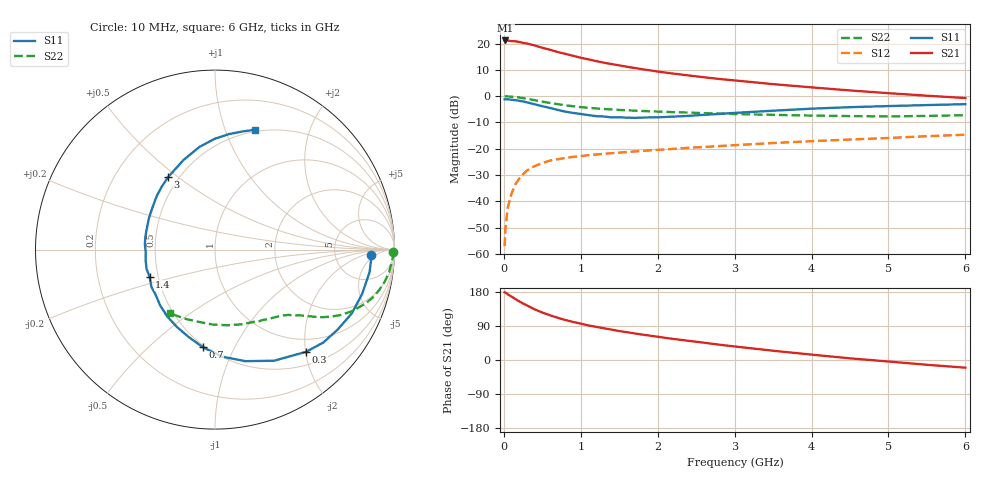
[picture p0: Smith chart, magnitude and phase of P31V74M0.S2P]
! SIEMENS Small Signal Semiconductors
! BFP181
! Si NPN RF Bipolar Junction Transistor in SOT143
! VCE = 1.75 V  IC = 4 mA
! Common Emitter S-Parameters:  March  1996
# GHz  S  MA  R  50
!  f  S11  S21  S12  S22
! GHz  MAG  ANG  MAG  ANG  MAG  ANG  MAG  ANG
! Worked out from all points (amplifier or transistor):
!   36 points, 10 MHz to 6 GHz, reference 50 ohm
!   highest |S21| = 21.2 dB at 20 MHz (marker M1)
!   |S21| within 3 dB of that: start of sweep to 527.5 MHz
!   unconditionally stable (mu >= 1): 1.756 GHz to end of sweep
!   at 250 MHz: K = 0.19, MSG = 25.0 dB, |S12| = -29.7 dB
!   at 1.4 GHz: K = 0.88, MSG = 17.0 dB, |S12| = -21.7 dB
!   at 6 GHz: K = 1.08, MAG = 5.3 dB, |S12| = -14.7 dB
!   S11 on the Smith chart (normalised r, x): 10 MHz: 14, -3; 300 MHz: 0.74, -2.01; 700 MHz: 0.49, -0.76; 1.4 GHz: 0.45, -0.16; 3 GHz: 0.44, +0.46; 6 GHz: 0.48, +1.28
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0.01  0.8713 -1.8  11.41 178.8  0.0014 78.2  0.9923 -0.7
0.02  0.8719 -3.4  11.48 177.9  0.0029 85.8  0.995 -1.4
0.05  0.8703 -8.4  11.45 173.5  0.0075 86.7  0.988 -3.7
0.15  0.841 -25.0  11.06 160.8  0.0211 75.2  0.9622 -10.7
0.2  0.8158 -33.1  10.76 154.8  0.027 72.3  0.9419 -13.9
0.25  0.7949 -40.7  10.34 149.1  0.0326 68.1  0.9183 -16.9
0.3  0.7627 -48.3  10.05 144.1  0.0385 64.4  0.8926 -19.5
0.4  0.7013 -62.0  9.232 133.7  0.0466 58.0  0.8391 -24.1
0.5  0.6441 -74.8  8.324 125.3  0.0534 52.7  0.7876 -27.6
0.6  0.5976 -86.2  7.643 118.0  0.0595 48.9  0.7434 -30.2
0.7  0.5483 -97.1  6.915 111.4  0.0631 46.1  0.7048 -32.3
0.8  0.5077 -107.0  6.378 105.5  0.0667 43.7  0.6714 -33.9
0.9  0.4805 -116.2  5.866 100.5  0.07 41.5  0.6426 -35.3
1.1  0.4365 -134.4  5.018 91.3  0.0755 38.7  0.6009 -37.6
1.4  0.3949 -157.4  4.083 80.2  0.0822 36.2  0.5587 -40.8
1.8  0.3917 175.7  3.257 67.0  0.0907 34.8  0.5223 -44.8
2.2  0.408 154.3  2.69 55.7  0.0993 33.1  0.4971 -49.9
3  0.4807 123.1  1.994 35.7  0.1169 30.1  0.4572 -61.7
3.5  0.529 109.4  1.694 24.5  0.1283 27.9  0.4415 -70.6
4.5  0.6177 90.1  1.285 4.4  0.1497 22.3  0.4179 -91.6
5.5  0.6771 76.6  1.021 -12.6  0.1732 17.4  0.4208 -114.1
6  0.7049 71.4  0.921 -20.3  0.1848 13.9  0.4348 -125.5
